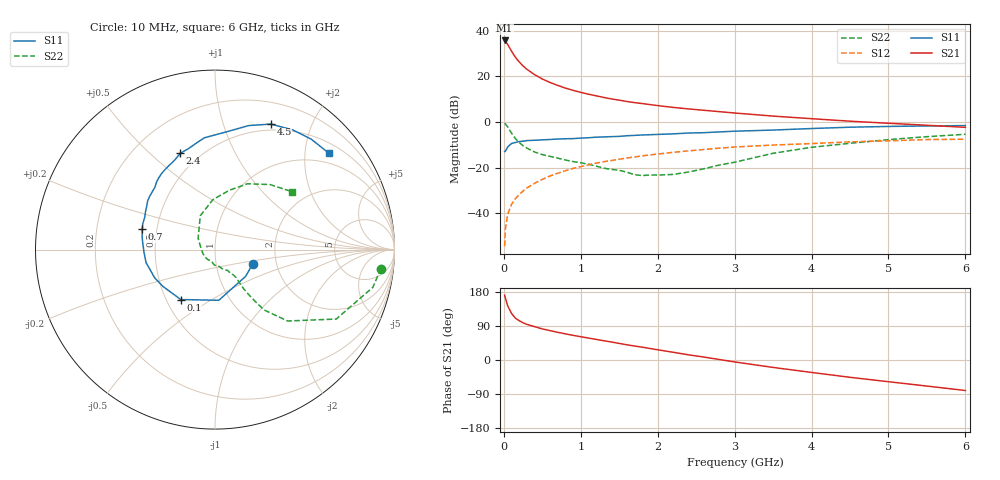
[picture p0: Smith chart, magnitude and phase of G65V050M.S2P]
! SIEMENS Small Signal Semiconductors
! BFG193
! Si NPN RF Bipolar Junction Transistor in SOT223
! VCE = 5 V  IC = 50 mA
! Common Emitter S-Parameters:  August  1996
# GHz  S  MA  R  50
!  f  S11  S21  S12  S22
! GHz  MAG  ANG  MAG  ANG  MAG  ANG  MAG  ANG
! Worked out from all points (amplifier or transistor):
!   36 points, 10 MHz to 6 GHz, reference 50 ohm
!   highest |S21| = 35.7 dB at 10 MHz (marker M1)
!   |S21| within 3 dB of that: start of sweep to 71.36 MHz
!   unconditionally stable (mu >= 1): 450.3 MHz to 2.36 GHz
!   at 250 MHz: K = 0.91, MSG = 27.4 dB, |S12| = -30.3 dB
!   at 1.4 GHz: K = 1.04, MAG = 12.2 dB, |S12| = -16.9 dB
!   at 6 GHz: K = 0.89, MSG = 2.6 dB, |S12| = -7.6 dB
!   S11 on the Smith chart (normalised r, x): 10 MHz: 1.50, -0.26; 100 MHz: 0.59, -0.37; 700 MHz: 0.41, +0.11; 2.4 GHz: 0.39, +0.63; 4.5 GHz: 0.43, +1.45; 6 GHz: 0.73, +2.53
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0.01  0.2248 -21.5  60.77 171.0  0.0019 87.7  0.9303 -6.5
0.02  0.2266 -41.2  58.55 163.6  0.0045 82.9  0.9046 -13.4
0.05  0.2833 -85.7  49.73 142.8  0.0095 73.5  0.7785 -29.8
0.1  0.3372 -124.4  35.43 122.9  0.0157 67.5  0.5675 -44.5
0.15  0.3548 -144.5  26.06 110.4  0.0208 66.4  0.433 -50.9
0.2  0.3712 -154.8  20.54 103.6  0.0256 68.0  0.3561 -52.4
0.25  0.3789 -163.1  16.79 98.2  0.0307 68.7  0.2996 -53.4
0.3  0.3908 -169.1  14.21 94.0  0.0358 69.5  0.2674 -53.8
0.4  0.3957 -177.5  10.83 88.0  0.0453 69.7  0.2191 -53.4
0.5  0.4046 174.6  8.703 82.1  0.0551 68.7  0.1922 -53.0
0.6  0.412 170.1  7.311 77.5  0.0656 67.6  0.1758 -54.0
0.7  0.4211 164.4  6.299 73.1  0.075 66.4  0.1611 -55.9
0.9  0.4309 155.3  4.913 65.1  0.0959 62.8  0.1353 -59.0
1.1  0.4498 147.9  4.043 57.9  0.115 59.3  0.1185 -67.9
1.3  0.4692 141.0  3.433 50.8  0.1345 55.1  0.0972 -75.9
1.6  0.498 130.8  2.797 40.1  0.1622 48.4  0.0791 -97.1
2.2  0.5471 114.2  2.08 20.4  0.2156 34.9  0.0708 -161.0
2.4  0.5705 109.8  1.926 13.7  0.2321 30.7  0.0799 172.0
3.5  0.6629 83.6  1.341 -19.6  0.3113 3.7  0.2055 113.5
4.5  0.7654 66.0  1.037 -45.7  0.3657 -16.2  0.3402 76.4
5.5  0.8162 48.9  0.844 -68.8  0.411 -39.5  0.475 49.7
6  0.8309 40.4  0.76 -80.5  0.4172 -53.0  0.5364 37.0
